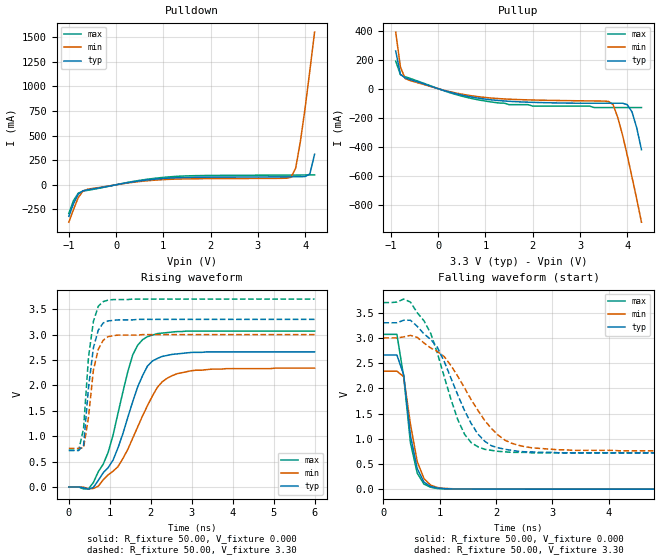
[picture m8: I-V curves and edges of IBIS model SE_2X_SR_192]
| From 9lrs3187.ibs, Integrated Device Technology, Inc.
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|   Model SE_2X_SR_192
[Model]   SE_2X_SR_192
Model_type   Output
Polarity   Inverting
Vmeas =   1.50V
Cref =   5.00pF
Rref =  50.000
Vref =   1.50V
C_comp   3.40pF   2.85pF   3.95pF
[Temperature Range]   27.00   70.00   0.000
[Voltage Range]   3.30V   3.00V   3.70V
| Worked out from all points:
|   slope of the pulldown table from 0 to 0.495 V, typ, clamps not added: 12.7 ohm
|   slope of the pullup table from 0 to 0.495 V, typ, clamps not added: 11.3 ohm
|   rising waveform, R_fixture 50.00, V_fixture 0.000: 20-80 % time 685ps typ, 847ps min, 582ps max; typ from 0 V to 2.66 V
|   rising waveform, R_fixture 50.00, V_fixture 3.30: 20-80 % time 211ps typ, 226ps min, 199ps max; typ from 0.72 V to 3.3 V
|   falling waveform, R_fixture 50.00, V_fixture 0.000: 20-80 % time 203ps typ, 223ps min, 213ps max; typ from 2.66 V to 0 V
|   falling waveform, R_fixture 50.00, V_fixture 3.30: 20-80 % time 625ps typ, 782ps min, 513ps max; typ from 3.3 V to 0.72 V
[Pulldown]
| voltage   I(typ)   I(min)   I(max)
|  -3.30   -4.16A   -4.01A   -4.26A
|  -3.10   -3.82A   -3.69A   -3.90A
|  -2.90   -3.48A   -3.37A   -3.55A
|  -2.70   -3.14A   -3.05A   -3.20A
|  -2.50   -2.80A   -2.72A   -2.85A
|  -2.30   -2.46A   -2.41A   -2.50A
|  -2.10   -2.12A   -2.09A   -2.15A
|  -1.90   -1.79A   -1.77A   -1.80A
|  -1.70   -1.45A   -1.45A   -1.45A
|  -1.50   -1.12A   -1.14A   -1.11A
-1V       -320mA     -380mA     -290mA
-900mV    -190mA     -250mA     -160mA
-800mV    -94.75mA   -130mA     -84.77mA
-700mV    -60.71mA   -64.75mA   -65.52mA
-600mV    -51.06mA   -45.2mA    -56.5mA
1.2V      69.5mA     56.57mA    82.87mA
3.7V      80.56mA    75.15mA    98.32mA
3.8V      80.96mA    170mA      98.58mA
3.9V      81.72mA    440mA      98.88mA
4V        83.73mA    780mA      99.22mA
4.1V      110mA      1.16A      99.62mA
4.2V      310mA      1.55A      100mA
|   4.30   0.66A   1.95A   0.10A
|   4.50   1.46A   2.77A   0.11A
|   4.70   2.32A   3.60A   0.58A
|   4.90   3.19A   4.43A   1.41A
|   5.10   4.07A   5.27A   2.30A
|   5.30   4.96A   6.12A   3.20A
|   5.50   5.85A   6.96A   4.12A
|   5.70   6.75A   7.81A   5.04A
|   5.90   7.65A   8.66A   5.97A
|   6.10   8.55A   9.52A   6.90A
|   6.60   10.81A   11.65A   9.23A
[Pullup]
| voltage   I(typ)   I(min)   I(max)
|  -3.30   10.68A   10.27A   10.94A
|  -3.10   9.79A   9.43A   10.01A
|  -2.90   8.89A   8.58A   9.09A
|  -2.70   7.99A   7.73A   8.16A
|  -2.50   7.10A   6.88A   7.23A
|  -2.30   6.20A   6.04A   6.31A
|  -2.10   5.31A   5.20A   5.38A
|  -1.90   4.43A   4.36A   4.47A
|  -1.70   3.54A   3.53A   3.55A
|  -1.50   2.67A   2.70A   2.64A
|  -1.00   0.59A   0.73A   0.50A
-900mV    260mA      390mA      190mA
-800mV    98.15mA    150mA      96.76mA
-700mV    74.35mA    69.94mA    82.79mA
-600mV    63.81mA    56.49mA    71.52mA
500mV     -44.25mA   -37.82mA   -51.47mA
1.5V      -86.95mA   -72.42mA   -110mA
3.5V      -100mA     -85.41mA   -130mA
3.7V      -100mA     -110mA     -130mA
3.9V      -100mA     -320mA     -130mA
4.1V      -160mA     -610mA     -130mA
4.2V      -270mA     -760mA     -130mA
4.3V      -420mA     -920mA     -130mA
|   4.50   -0.73A   -1.22A   -0.15A
|   4.70   -1.06A   -1.54A   -0.40A
|   4.90   -1.39A   -1.86A   -0.73A
|   5.10   -1.72A   -2.17A   -1.06A
|   5.30   -2.06A   -2.49A   -1.41A
|   5.50   -2.40A   -2.81A   -1.75A
|   5.70   -2.74A   -3.13A   -2.10A
|   5.90   -3.07A   -3.46A   -2.45A
|   6.10   -3.41A   -3.78A   -2.80A
|   6.60   -4.27A   -4.58A   -3.68A
[Ramp]
| variable   typ   min   max
dV/dt_r   1.60/0.68n   1.40/0.84n   1.84/0.57n
dV/dt_f   1.55/0.62n   1.34/0.77n   1.79/0.50n
R_load = 50.00
[Rising Waveform]
R_fixture = 50.00
V_fixture = 0.000
V_fixture_min = 0.000
V_fixture_max = 0.000
| time   V(typ)   V(min)   V(max)
0s        0V         1.34uV     0V
480ps     -43.38mV   -36.81mV   -36.84mV
840ps     280mV      140mV      450mV
1.08ns    530mV      310mV      1.02V
1.56ns    1.68V      960mV      2.6V
1.8ns     2.19V      1.4V       2.9V
1.92ns    2.38V      1.6V       2.96V
2.16ns    2.53V      1.96V      3.02V
2.64ns    2.62V      2.23V      3.06V
6ns       2.66V      2.34V      3.07V
[Rising Waveform]
R_fixture = 50.00
V_fixture = 3.30
V_fixture_min = 3.00
V_fixture_max = 3.70
| time   V(typ)   V(min)   V(max)
0s        720mV      760mV      720mV
240ps     720mV      760mV      720mV
360ps     820mV      770mV      1.15V
480ps     1.95V      1.37V      2.55V
600ps     2.74V      2.3V       3.26V
720ps     3.09V      2.71V      3.56V
840ps     3.23V      2.89V      3.65V
960ps     3.27V      2.96V      3.68V
1.2ns     3.29V      2.99V      3.69V
6ns       3.3V       3V         3.7V
[Falling Waveform]
R_fixture = 50.00
V_fixture = 0.000
V_fixture_min = 0.000
V_fixture_max = 0.000
| time   V(typ)   V(min)   V(max)
0s        2.66V      2.34V      3.07V
240ps     2.66V      2.34V      3.07V
360ps     2.27V      2.23V      2.23V
480ps     1.06V      1.29V      920mV
600ps     410mV      550mV      320mV
720ps     140mV      210mV      100mV
840ps     52.27mV    79mV       37.5mV
960ps     23.77mV    32.48mV    11.83mV
1.32ns    3.61mV     5.56mV     2.9mV
6ns       0V         1.85uV     0V
[Falling Waveform]
R_fixture = 50.00
V_fixture = 3.30
V_fixture_min = 3.00
V_fixture_max = 3.70
| time   V(typ)   V(min)   V(max)
0s        3.3V       3V         3.7V
360ps     3.35V      3.02V      3.77V
720ps     3.08V      2.9V       3.34V
960ps     2.81V      2.73V      2.69V
1.32ns    1.87V      2.24V      1.38V
1.44ns    1.56V      2.01V      1.09V
1.68ns    1.09V      1.56V      840mV
2.04ns    820mV      1.07V      750mV
2.52ns    740mV      840mV      730mV
6ns       720mV      760mV      720mV
